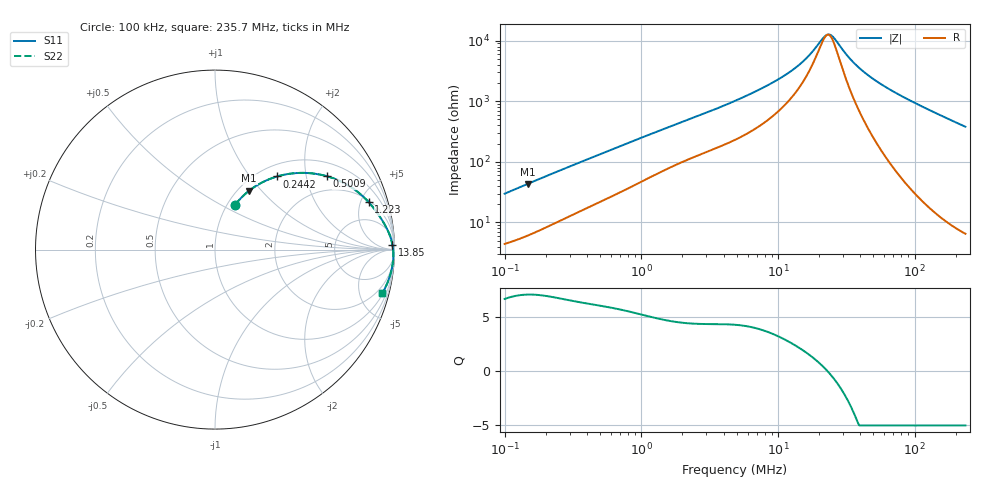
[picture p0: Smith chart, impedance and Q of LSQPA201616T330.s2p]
! LSQPA201616T330  S-PARAMETER MODEL  ( General Type )
! Model Generated by TAIYO YUDEN Corporation (http://www.ty-top.com)
! Version 2.0
! TAIYO YUDEN Control No. 100810NF25SB-FKC
! Copyright(c) 2007 TAIYO YUDEN CO.,LTD. All Rights Reserved.
! Product Description (link to TY-COMPAS)
! https://ds.yuden.co.jp/TYCOMPAS/or/detail?pn=LSQPA201616T330K&u=M
! Products Name : Inductors
! Characteristics :
!  Inductance : 33 uH , SRF(min) : 14 MHz , DC Resistance(max) : 3.64 Ohm
!  Rated Current : Saturation :220 mA , Temp Rise : 220 mA (40 degC)
!  Case Size : 2.0 x 1.6 / 0.079 x 0.063 [mm/inch] , Thickness : 1.6 / 0.063 [mm/inch]
!  (Conditions: Temperature = 25 degC , DC Bias Current/Voltage = 0A / 0V)
! External Node Assignments :
!  1  o---GGG---o  2
! GND o---------o GND
! Frequency Range : 0.1MHz  -  235.669543MHz  [ 402 STEP ]
# MHz S RI R 50
! Freq[MHz].  S11 Real  S11 Imag  S21 Real  S21 Imag  S12 Real  S12 Imag  S22 Real  S22 Imag
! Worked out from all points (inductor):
!   401 points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, 100 kHz to 235.7 MHz, reference 50 ohm
!   read as one part in series: L = 46.5 uH near 104 kHz
!   highest Q = 7.07 at 147.4 kHz (marker M1), where L = 46.2 uH
!   self-resonance near 22.94 MHz
!   S11 on the Smith chart (normalised r, x): 100 kHz: 1.09, +0.59; 244.2 kHz: 1.20, +1.38; 500.9 kHz: 1.44, +2.64; 1.223 MHz: 2.18, +5.85; 13.85 MHz: 31, +69; 235.7 MHz: 1.13, -7.59
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0.1  0.1128 0.2502  0.8872 -0.2502  0.8872 -0.2502  0.1128 0.2502
0.14744  0.1894 0.3274  0.8106 -0.3274  0.8106 -0.3274  0.1894 0.3274
0.244239  0.3468 0.4077  0.6532 -0.4077  0.6532 -0.4077  0.3468 0.4077
0.367165  0.5042 0.4272  0.4958 -0.4272  0.4958 -0.4272  0.5042 0.4272
0.500902  0.6226 0.409  0.3774 -0.409  0.3774 -0.409  0.6226 0.409
0.782817  0.7635 0.3444  0.2365 -0.3444  0.2365 -0.3444  0.7635 0.3444
1.223398  0.8565 0.264  0.1435 -0.264  0.1435 -0.264  0.8565 0.264
1.348099  0.8711 0.2473  0.1289 -0.2473  0.1289 -0.2473  0.8711 0.2473
2.367084  0.9303 0.1651  0.0697 -0.1651  0.0697 -0.1651  0.9303 0.1651
4.854581  0.9696 0.091  0.0304 -0.091  0.0304 -0.091  0.9696 0.091
9.035163  0.9842 0.0466  0.0158 -0.0466  0.0158 -0.0466  0.9842 0.0466
13.84882  0.9888 0.0238  0.0112 -0.0238  0.0112 -0.0238  0.9888 0.0238
17.8243  0.9906 0.012  0.00936 -0.012  0.00936 -0.012  0.9906 0.012
22.06739  0.9919 0.00216  0.00811 -0.00216  0.00811 -0.00216  0.9919 0.00216
24.3167  0.9924 -0.00238  0.00763 0.00238  0.00763 0.00238  0.9924 -0.00238
26.28014  0.9927 -0.00608  0.00728 0.00608  0.00728 0.00608  0.9927 -0.00608
33.17392  0.9935 -0.0178  0.00647 0.0178  0.00647 0.0178  0.9935 -0.0178
38.74743  0.9938 -0.0264  0.00619 0.0264  0.00619 0.0264  0.9938 -0.0264
48.91162  0.9937 -0.0408  0.00634 0.0408  0.00634 0.0408  0.9937 -0.0408
65.44454  0.9922 -0.0624  0.00784 0.0624  0.00784 0.0624  0.9922 -0.0624
117.1645  0.9811 -0.1234  0.0189 0.1234  0.0189 0.1234  0.9811 -0.1234
235.6695  0.9315 -0.2442  0.0685 0.2442  0.0685 0.2442  0.9315 -0.2442
